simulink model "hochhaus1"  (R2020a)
settings: Solver=ode45  StartTime=0.0  StopTime=2  MaxStep=1e-3  RelTol=1e-3  EnableMultiTasking=on

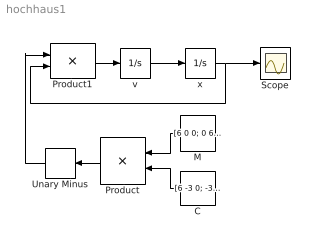
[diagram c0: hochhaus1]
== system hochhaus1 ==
  note: .
  C : Constant  Value=[6 -3 0; -3 4 -1; 0 -1 1]*1e6  VectorParams1D=off
  M : Constant  Value=[6 0 0; 0 6 0; 0 0 1]*1e3  VectorParams1D=off
  Product : Product  Inputs=/*  Multiplication=Matrix(*)  InputSameDT=on  SaturateOnIntegerOverflow=on
  Product1 : Product  Multiplication=Matrix(*)  InputSameDT=on  SaturateOnIntegerOverflow=on
  Scope : Scope
  Unary Minus : UnaryMinus
  v : Integrator  InitialCondition=[0; 0; 10]
  x : Integrator  InitialCondition=[0; 0; 0]
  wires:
  v/1 -> x/1
  x/1 -> Scope/1, Product1/2
  M/1 -> Product/1
  C/1 -> Product/2
  Product1/1 -> v/1
  Unary Minus/1 -> Product1/1
  Product/1 -> Unary Minus/1
